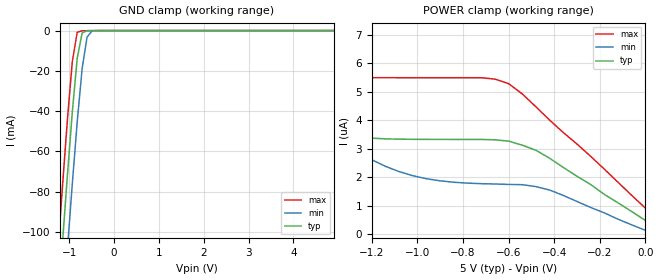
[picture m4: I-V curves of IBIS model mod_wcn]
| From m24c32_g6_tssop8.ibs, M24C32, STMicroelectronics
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|   Model mod_wcn
[Model]   mod_wcn
Model_type Input
Vinl   =   1.500V
Vinh   =   3.500V
C_comp   2.119pF   2.023pF   2.323pF
[Temperature Range]   25.0000   0.1250k   -40.0000
[Voltage Range]   5.0000V   4.5000V   5.5000V
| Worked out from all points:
|   GND clamp passes 1 mA (typ) near -0.70 V on its own axis
[GND_clamp]
|Voltage   I(typ)   I(min)   I(max)
-5V       -1.381A    -1.415A    -1.356A
-1.26V    -140.4mA   -177.6mA   -112.3mA
-1.15V    -105.9mA   -143.1mA   -77.85mA
-1.04V    -72.4mA    -109.2mA   -44.81mA
-930mV    -40.73mA   -76.34mA   -15.55mA
-820mV    -13.84mA   -45.44mA   -867.4uA
-710mV    -1.105mA   -18.88mA   -97.48uA
-600mV    -55.62uA   -3.201mA   -59.79uA
-490mV    -14.19uA   -211.3uA   -30.28uA
4.9V      3.327uA    1.881uA    5.49uA
[POWER_clamp]
|Voltage   I(typ)   I(min)   I(max)
-4.98V    62.36uA    50.65uA    77.93uA
-1.98V    8.751uA    7.146uA    10.26uA
-1.86V    7.195uA    6.878uA    8.441uA
-1.74V    5.793uA    6.549uA    7.082uA
-1.68V    5.221uA    6.238uA    6.585uA
-1.56V    4.342uA    5.09uA     5.918uA
-1.38V    3.608uA    3.61uA     5.542uA
-1.08V    3.337uA    2.198uA    5.49uA
-720mV    3.327uA    1.777uA    5.49uA
-600mV    3.268uA    1.751uA    5.28uA
-420mV    2.665uA    1.553uA    4.002uA
0V        487.1nA    142.1nA    919.3nA
